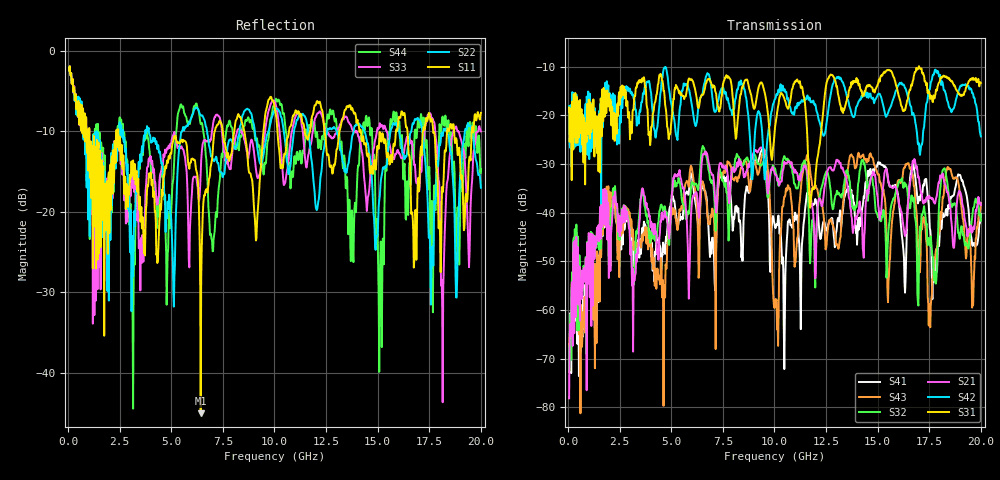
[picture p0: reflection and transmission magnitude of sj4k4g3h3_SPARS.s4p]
! FILE: E:\users\goganessyan\GBX_Backplane\FR408_backplane\1m_OUTBOUND_NEXT\sj4k4g3h3_SPARS.s4p
# MHZ S RI R 50.00
! FREQ  S11  S12  S13  S14
!  S21  S22  S23  S24
!  S31  S32  S33  S34
!  S41  S42  S43  S44
!  REAL  IMAG  REAL  IMAG  REAL  IMAG  REAL  IMAG
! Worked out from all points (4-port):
!   799 points, 50 MHz to 20 GHz, reference 50 ohm
!   strongest paths, dB at 50 MHz, 5.025 GHz, 10.03 GHz, 15.03 GHz, 20 GHz:
!     S31: -18.4, -20.3, -22.5, -13.5, -13.3
!     S42: -18.1, -18.3, -16.6, -15.6, -24.3
!     S21: -78.1, -36.2, -32.2, -38.5, -38.4
!     S32: -67.4, -36.3, -30.8, -41.0, -41.6
!     S43: -68.6, -40.3, -59.0, -32.2, -38.0
!     S41: -72.7, -37.2, -42.9, -29.6, -40.2
!   lowest |S11| = -45.0 dB at 6.425 GHz (marker M1), VSWR 1.01, Z = 49.7 + j0.483 ohm
!   |S11| at or under -10 dB: 1.027 GHz to 2.343 GHz (1.316 GHz wide, 78.1 % of centre); 2.43 GHz to 7.1 GHz (4.67 GHz wide, 98 % of centre); 14.18 GHz to 15.89 GHz (1.703 GHz wide, 11.3 % of centre)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
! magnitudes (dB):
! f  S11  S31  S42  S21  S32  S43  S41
! 50 MHz  -2.5  -18.4  -18.1  -78.1  -67.4  -68.6  -72.7
! 1.775 GHz  -17.6  -20.2  -14.7  -35.1  -35.1  -35.7  -36.0
! 3.15 GHz  -13.6  -18.9  -15.7  -68.5  -52.0  -44.1  -46.0
! 6.425 GHz  -45.0  -16.2  -16.3  -33.4  -29.2  -36.8  -36.7
! 16.43 GHz  -9.6  -16.9  -15.5  -41.0  -35.0  -29.9  -41.9
! 17.52 GHz  -8.1  -16.1  -14.7  -37.0  -45.7  -62.8  -43.2
! 20 GHz  -7.7  -13.3  -24.3  -38.4  -41.6  -38.0  -40.2
